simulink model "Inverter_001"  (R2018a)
settings: Solver=FixedStepDiscrete  StartTime=0.0  StopTime=inf  RelTol=1e-3  EnableMultiTasking=on
PreLoadFcn:
  | Sample_Time
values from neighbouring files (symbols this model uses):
  C_filt = 9.2e-6    (= 9.2e-06)    [master5.m]    (also in Sample_Time.m = 1.175e-06)
  Kcp = 5 /2    (= 2.5)    [master5.m]    (also in Parametri_final.m = Kcp_rac*20; Sample_Time.m = 8.8)
  Kcp0 = 5 /2    (= 2.5)    [master5.m]    (also in Parametri_final.m = Kc0p_rac*20; Sample_Time.m = 8.8)
  Kvp = 1    [master5.m]    (also in Parametri_final.m = 0.06652; Sample_Time.m = 2.4)
  Kvp0 = 1    [master5.m]    (also in Parametri_final.m = 0.06652; Sample_Time.m = 2.4)
  L_filt = 1e-3    (= 0.001)    [master5.m]    (also in Sample_Time.m = 0.01)
  Tcontrol = 5e-5     *2    (= 0.0001)    [Sample_Time.m]
  Tmeasure = 5e-5    (= 5e-05)    [Sample_Time.m]
  w = 2*pi*50    (= 314.159265359)    [master5.m]    (also in Parametri_final.m = 314.1592)
undefined symbols (not defined in the file or in its folder): A, ADCIN0, ADCIN1, ADCINA0, ADCINB0, bit, C_filtEST, CC_Tci, CC_Tci0, CC_Tcr, Compare, Control, conversion, DCAEVT1, DCAEVT1FILT, Digital, Down, ended, Event, Filtered, GPTRIP1SEL, GPTRIP2SEL, input, Module, of, Single, start, Trip, TZ1, TZ2, Up, VC_Tci, VC_Tci0, VC_Tcr, version, Zone
libraries: tiiqmathlib x92, etargetslib x20, c2802xlib x13, c2837xDlib x7, c28xdmclib x1
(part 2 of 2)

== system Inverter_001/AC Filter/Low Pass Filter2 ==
  Input : Inport
  TimeConstant : Inport  Port=2
  IQN1 x IQN2 : tiiqmathlib/IQN1 x IQN2  Q=10
  Sum1 : Sum  Inputs=|+-  AccumDataTypeStr=single
  Sum2 : Sum  Inputs=|++  AccumDataTypeStr=single
  Sum3 : Sum  Inputs=|+-
  Unit Delay : UnitDelay  SampleTime=-1
  Unit Delay1 : UnitDelay  SampleTime=-1
  Output : Outport
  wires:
  Input/1 -> Sum3/1, Sum1/1
  IQN1 x IQN2/1 -> Sum1/2  "TcState"
  Sum1/1 -> Sum3/2, Unit Delay/1  "HighPassFilterOutput"
  Sum2/1 -> Unit Delay1/1, IQN1 x IQN2/2  "state"
  Unit Delay/1 -> Sum2/1
  TimeConstant/1 -> IQN1 x IQN2/1  "tc"
  Unit Delay1/1 -> Sum2/2
  Sum3/1 -> Output/1  "HighPassFilterOutput"

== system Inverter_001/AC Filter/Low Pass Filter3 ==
  Input : Inport
  TimeConstant : Inport  Port=2
  IQN1 x IQN2 : tiiqmathlib/IQN1 x IQN2  Q=10
  Sum1 : Sum  Inputs=|+-  AccumDataTypeStr=single
  Sum2 : Sum  Inputs=|++  AccumDataTypeStr=single
  Sum3 : Sum  Inputs=|+-
  Unit Delay : UnitDelay  SampleTime=-1
  Unit Delay1 : UnitDelay  SampleTime=-1
  Output : Outport
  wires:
  Sum3/1 -> Output/1  "HighPassFilterOutput"
  Unit Delay1/1 -> Sum2/2
  TimeConstant/1 -> IQN1 x IQN2/1  "tc"
  Unit Delay/1 -> Sum2/1
  Sum2/1 -> IQN1 x IQN2/2, Unit Delay1/1  "state"
  Sum1/1 -> Unit Delay/1, Sum3/2  "HighPassFilterOutput"
  IQN1 x IQN2/1 -> Sum1/2  "TcState"
  Input/1 -> Sum1/1, Sum3/1

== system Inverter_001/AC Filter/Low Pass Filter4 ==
  Input : Inport
  TimeConstant : Inport  Port=2
  IQN1 x IQN2 : tiiqmathlib/IQN1 x IQN2  Q=10
  Sum1 : Sum  Inputs=|+-  AccumDataTypeStr=single
  Sum2 : Sum  Inputs=|++  AccumDataTypeStr=single
  Sum3 : Sum  Inputs=|+-
  Unit Delay : UnitDelay  SampleTime=-1
  Unit Delay1 : UnitDelay  SampleTime=-1
  Output : Outport
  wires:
  Input/1 -> Sum3/1, Sum1/1
  IQN1 x IQN2/1 -> Sum1/2  "TcState"
  Sum1/1 -> Sum3/2, Unit Delay/1  "HighPassFilterOutput"
  Sum2/1 -> Unit Delay1/1, IQN1 x IQN2/2  "state"
  Unit Delay/1 -> Sum2/1
  TimeConstant/1 -> IQN1 x IQN2/1  "tc"
  Unit Delay1/1 -> Sum2/2
  Sum3/1 -> Output/1  "HighPassFilterOutput"

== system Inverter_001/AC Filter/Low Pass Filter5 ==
  Input : Inport
  TimeConstant : Inport  Port=2
  IQN1 x IQN2 : tiiqmathlib/IQN1 x IQN2  Q=10
  Sum1 : Sum  Inputs=|+-  AccumDataTypeStr=single
  Sum2 : Sum  Inputs=|++  AccumDataTypeStr=single
  Sum3 : Sum  Inputs=|+-
  Unit Delay : UnitDelay  SampleTime=-1
  Unit Delay1 : UnitDelay  SampleTime=-1
  Output : Outport
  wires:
  Sum3/1 -> Output/1  "HighPassFilterOutput"
  Unit Delay1/1 -> Sum2/2
  TimeConstant/1 -> IQN1 x IQN2/1  "tc"
  Unit Delay/1 -> Sum2/1
  Sum2/1 -> IQN1 x IQN2/2, Unit Delay1/1  "state"
  Sum1/1 -> Unit Delay/1, Sum3/2  "HighPassFilterOutput"
  IQN1 x IQN2/1 -> Sum1/2  "TcState"
  Input/1 -> Sum1/1, Sum3/1

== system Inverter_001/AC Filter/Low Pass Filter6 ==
  Input : Inport
  TimeConstant : Inport  Port=2
  IQN1 x IQN2 : tiiqmathlib/IQN1 x IQN2  Q=10
  Sum1 : Sum  Inputs=|+-  AccumDataTypeStr=single
  Sum2 : Sum  Inputs=|++  AccumDataTypeStr=single
  Sum3 : Sum  Inputs=|+-
  Unit Delay : UnitDelay  SampleTime=-1
  Unit Delay1 : UnitDelay  SampleTime=-1
  Output : Outport
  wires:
  Input/1 -> Sum3/1, Sum1/1
  IQN1 x IQN2/1 -> Sum1/2  "TcState"
  Sum1/1 -> Sum3/2, Unit Delay/1  "HighPassFilterOutput"
  Sum2/1 -> Unit Delay1/1, IQN1 x IQN2/2  "state"
  Unit Delay/1 -> Sum2/1
  TimeConstant/1 -> IQN1 x IQN2/1  "tc"
  Unit Delay1/1 -> Sum2/2
  Sum3/1 -> Output/1  "HighPassFilterOutput"

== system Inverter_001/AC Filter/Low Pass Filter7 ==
  Input : Inport
  TimeConstant : Inport  Port=2
  IQN1 x IQN2 : tiiqmathlib/IQN1 x IQN2  Q=10
  Sum1 : Sum  Inputs=|+-  AccumDataTypeStr=single
  Sum2 : Sum  Inputs=|++  AccumDataTypeStr=single
  Sum3 : Sum  Inputs=|+-
  Unit Delay : UnitDelay  SampleTime=-1
  Unit Delay1 : UnitDelay  SampleTime=-1
  Output : Outport
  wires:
  Sum3/1 -> Output/1  "HighPassFilterOutput"
  Unit Delay1/1 -> Sum2/2
  TimeConstant/1 -> IQN1 x IQN2/1  "tc"
  Unit Delay/1 -> Sum2/1
  Sum2/1 -> IQN1 x IQN2/2, Unit Delay1/1  "state"
  Sum1/1 -> Unit Delay/1, Sum3/2  "HighPassFilterOutput"
  IQN1 x IQN2/1 -> Sum1/2  "TcState"
  Input/1 -> Sum1/1, Sum3/1

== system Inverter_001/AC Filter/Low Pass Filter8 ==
  Input : Inport
  TimeConstant : Inport  Port=2
  IQN1 x IQN2 : tiiqmathlib/IQN1 x IQN2  Q=10
  Sum1 : Sum  Inputs=|+-  AccumDataTypeStr=single
  Sum2 : Sum  Inputs=|++  AccumDataTypeStr=single
  Sum3 : Sum  Inputs=|+-
  Unit Delay : UnitDelay  SampleTime=-1
  Unit Delay1 : UnitDelay  SampleTime=-1
  Output : Outport
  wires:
  Input/1 -> Sum3/1, Sum1/1
  IQN1 x IQN2/1 -> Sum1/2  "TcState"
  Sum1/1 -> Sum3/2, Unit Delay/1  "HighPassFilterOutput"
  Sum2/1 -> Unit Delay1/1, IQN1 x IQN2/2  "state"
  Unit Delay/1 -> Sum2/1
  TimeConstant/1 -> IQN1 x IQN2/1  "tc"
  Unit Delay1/1 -> Sum2/2
  Sum3/1 -> Output/1  "HighPassFilterOutput"

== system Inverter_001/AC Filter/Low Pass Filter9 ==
  Input : Inport
  TimeConstant : Inport  Port=2
  IQN1 x IQN2 : tiiqmathlib/IQN1 x IQN2  Q=10
  Sum1 : Sum  Inputs=|+-  AccumDataTypeStr=single
  Sum2 : Sum  Inputs=|++  AccumDataTypeStr=single
  Sum3 : Sum  Inputs=|+-
  Unit Delay : UnitDelay  SampleTime=-1
  Unit Delay1 : UnitDelay  SampleTime=-1
  Output : Outport
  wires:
  Sum3/1 -> Output/1  "HighPassFilterOutput"
  Unit Delay1/1 -> Sum2/2
  TimeConstant/1 -> IQN1 x IQN2/1  "tc"
  Unit Delay/1 -> Sum2/1
  Sum2/1 -> IQN1 x IQN2/2, Unit Delay1/1  "state"
  Sum1/1 -> Unit Delay/1, Sum3/2  "HighPassFilterOutput"
  IQN1 x IQN2/1 -> Sum1/2  "TcState"
  Input/1 -> Sum1/1, Sum3/1

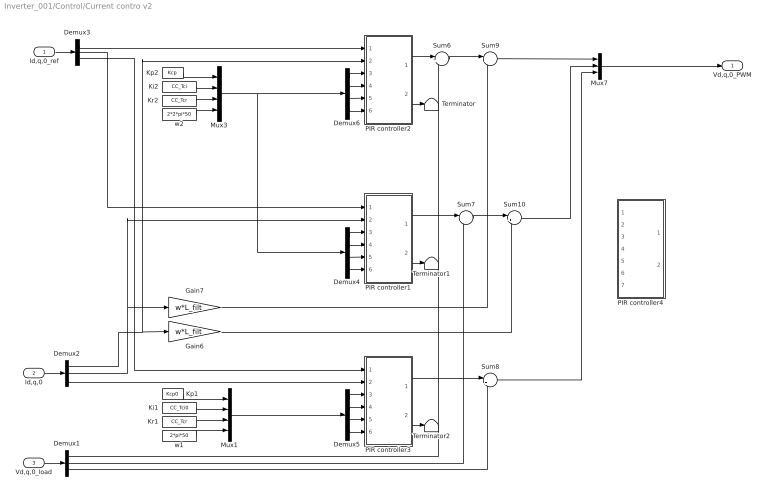
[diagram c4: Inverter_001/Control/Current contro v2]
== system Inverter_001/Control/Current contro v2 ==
  Id,q,0_ref : Inport
  Id,q,0 : Inport  Port=2
  Vd,q,0_load : Inport  Port=3
  Demux1 : Demux  Outputs=3
  Demux2 : Demux  Outputs=3
  Demux3 : Demux  Outputs=3
  Demux4 : Demux
  Demux5 : Demux
  Demux6 : Demux
  Gain6 : Gain  Gain=w*L_filt
  Gain7 : Gain  Gain=w*L_filt
  Ki1 : Constant  Value=CC_Tci0  OutDataTypeStr=fixdt(1,32,2^-10,0)  SampleTime=-1
  Ki2 : Constant  Value=CC_Tci  OutDataTypeStr=fixdt(1,32,2^-10,0)  SampleTime=-1
  Kp1 : Constant  Value=Kcp0  OutDataTypeStr=fixdt(1,32,2^-10,0)  SampleTime=-1
  Kp2 : Constant  Value=Kcp  OutDataTypeStr=fixdt(1,32,2^-10,0)  SampleTime=-1
  Kr1 : Constant  Value=CC_Tcr  OutDataTypeStr=fixdt(1,32,2^-10,0)  SampleTime=-1
  Kr2 : Constant  Value=CC_Tcr  OutDataTypeStr=fixdt(1,32,2^-10,0)  SampleTime=-1
  Mux1 : Mux
  Mux3 : Mux
  Mux7 : Mux  Inputs=3
  PIR controller1 : Subsystem
  PIR controller2 : Subsystem
  PIR controller3 : Subsystem
  PIR controller4 : Subsystem  Commented=on
  Sum{6..8,10} (4 alike) : Sum  Inputs=|++
  Sum9 : Sum  Inputs=|+-
  Terminator : Terminator
  Terminator1 : Terminator
  Terminator2 : Terminator
  w1 : Constant  Value=2*pi*50  OutDataTypeStr=fixdt(1,32,2^-10,0)  SampleTime=-1
  w2 : Constant  Value=2*2*pi*50  OutMin=[1e-4]  OutMax=[1000]  OutDataTypeStr=fixdt(1,32,2^-10,0)  SampleTime=-1
  Vd,q,0_PWM : Outport
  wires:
  Mux3/1 -> Demux4/1, Demux6/1
  w2/1 -> Mux3/4
  Kr2/1 -> Mux3/3
  Ki2/1 -> Mux3/2
  Kp2/1 -> Mux3/1
  Demux6/4 -> PIR controller2/6(w)
  Demux6/3 -> PIR controller2/5(Tr)
  Demux6/1 -> PIR controller2/3(Kp)
  Demux6/2 -> PIR controller2/4(Ti)
  Sum8/1 -> Mux7/3
  PIR controller1/1(Out1) -> Sum7/1
  Demux1/3 -> Sum8/2
  Demux3/3 -> PIR controller3/1(Reference)
  Demux2/3 -> PIR controller3/2(Measurement)
  PIR controller3/1(Out1) -> Sum8/1
  PIR controller2/1(Out1) -> Sum6/1
  Demux1/1 -> Sum6/2
  Demux1/2 -> Sum7/2
  Sum6/1 -> Sum9/1
  Sum9/1 -> Mux7/1
  Sum7/1 -> Sum10/1
  Sum10/1 -> Mux7/2
  Gain6/1 -> Sum10/2
  Gain7/1 -> Sum9/2
  Demux3/1 -> PIR controller2/1(Reference)
  Demux3/2 -> PIR controller1/1(Reference)
  Id,q,0/1 -> Demux2/1
  Id,q,0_ref/1 -> Demux3/1
  Vd,q,0_load/1 -> Demux1/1
  Demux2/2 -> PIR controller1/2(Measurement), Gain7/1
  Demux2/1 -> PIR controller2/2(Measurement), Gain6/1
  Demux5/1 -> PIR controller3/3(Kp)
  Demux5/2 -> PIR controller3/4(Ti)
  Demux5/3 -> PIR controller3/5(Tr)
  w1/1 -> Mux1/4
  Ki1/1 -> Mux1/2
  Kr1/1 -> Mux1/3
  Kp1/1 -> Mux1/1
  Mux1/1 -> Demux5/1
  Mux7/1 -> Vd,q,0_PWM/1
  Demux5/4 -> PIR controller3/6(w)
  Demux4/1 -> PIR controller1/3(Kp)
  Demux4/4 -> PIR controller1/6(w)
  Demux4/2 -> PIR controller1/4(Ti)
  Demux4/3 -> PIR controller1/5(Tr)
  PIR controller2/2(Error) -> Terminator/1
  PIR controller1/2(Error) -> Terminator1/1
  PIR controller3/2(Error) -> Terminator2/1

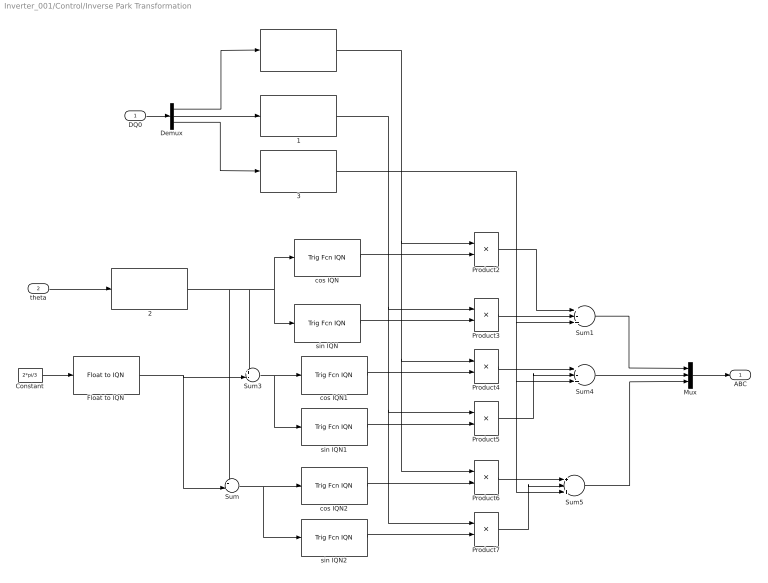
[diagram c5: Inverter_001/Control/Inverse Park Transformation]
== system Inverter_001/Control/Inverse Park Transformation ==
  DQ0 : Inport
  theta : Inport  Port=2
   {,1..3} (4 alike) : etargetslib/ 
  Constant : Constant  Value=2*pi/3  OutDataTypeStr=single
  Demux : Demux  Outputs=3
  Float to IQN : tiiqmathlib/Float to IQN  Q_value=10
  Mux : Mux  Inputs=3
  Product{2..7} (6 alike) : Product
  Sum : Sum  Inputs=++|
  Sum1 : Sum  Inputs=+-+
  Sum3 : Sum  Inputs=+-|
  Sum4 : Sum  Inputs=+-+
  Sum5 : Sum  Inputs=+-+
  cos IQN : tiiqmathlib/Trig Fcn IQN  functionOption=_IQcos
  cos IQN1 : tiiqmathlib/Trig Fcn IQN  functionOption=_IQcos
  cos IQN2 : tiiqmathlib/Trig Fcn IQN  functionOption=_IQcos
  sin IQN : tiiqmathlib/Trig Fcn IQN  functionOption=_IQsin
  sin IQN1 : tiiqmathlib/Trig Fcn IQN  functionOption=_IQsin
  sin IQN2 : tiiqmathlib/Trig Fcn IQN  functionOption=_IQsin
  ABC : Outport
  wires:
  " 2"/1 -> sin IQN/1, cos IQN/1, Sum3/1, Sum/1
  " 1"/1 -> Product7/1, Product5/1, Product3/1
  Mux/1 -> ABC/1
  Product2/1 -> Sum1/1
  Product3/1 -> Sum1/2
  sin IQN/1 -> Product3/2
  cos IQN/1 -> Product2/2
  Demux/2 -> " 1"/1
  Demux/1 -> " "/1
  theta/1 -> " 2"/1
  Demux/3 -> " 3"/1
  Constant/1 -> Float to IQN/1
  Float to IQN/1 -> Sum/2, Sum3/2
  " 3"/1 -> Sum5/3, Sum4/3, Sum1/3
  Sum3/1 -> sin IQN1/1, cos IQN1/1
  cos IQN1/1 -> Product4/2
  sin IQN1/1 -> Product5/2
  Product4/1 -> Sum4/1
  Product5/1 -> Sum4/2
  Sum4/1 -> Mux/2
  Sum/1 -> sin IQN2/1, cos IQN2/1
  " "/1 -> Product2/1, Product4/1, Product6/1
  cos IQN2/1 -> Product6/2
  sin IQN2/1 -> Product7/2
  Product6/1 -> Sum5/1
  Product7/1 -> Sum5/2
  Sum5/1 -> Mux/3
  DQ0/1 -> Demux/1
  Sum1/1 -> Mux/1

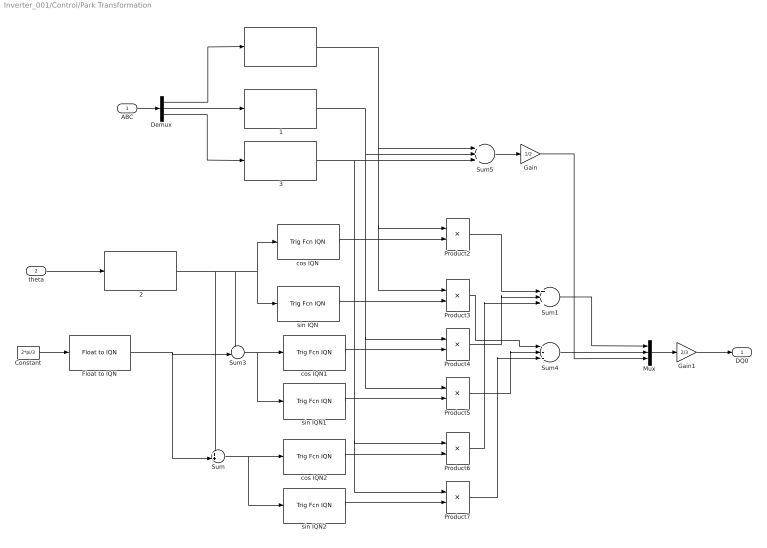
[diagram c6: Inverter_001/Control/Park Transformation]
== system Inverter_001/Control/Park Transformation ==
  ABC : Inport
  theta : Inport  Port=2
   {,1..3} (4 alike) : etargetslib/ 
  Constant : Constant  Value=2*pi/3  OutDataTypeStr=single
  Demux : Demux  Outputs=3
  Float to IQN : tiiqmathlib/Float to IQN  Q_value=10
  Gain : Gain  Gain=1/2  OutDataTypeStr=Inherit: Inherit via back propagation
  Gain1 : Gain  Gain=2/3  OutDataTypeStr=Inherit: Inherit via back propagation
  Mux : Mux  Inputs=3
  Product{2..7} (6 alike) : Product
  Sum : Sum  Inputs=++|
  Sum1 : Sum  Inputs=+++
  Sum3 : Sum  Inputs=+-|
  Sum4 : Sum  Inputs=---
  Sum5 : Sum  Inputs=+++
  cos IQN : tiiqmathlib/Trig Fcn IQN  functionOption=_IQcos
  cos IQN1 : tiiqmathlib/Trig Fcn IQN  functionOption=_IQcos
  cos IQN2 : tiiqmathlib/Trig Fcn IQN  functionOption=_IQcos
  sin IQN : tiiqmathlib/Trig Fcn IQN  functionOption=_IQsin
  sin IQN1 : tiiqmathlib/Trig Fcn IQN  functionOption=_IQsin
  sin IQN2 : tiiqmathlib/Trig Fcn IQN  functionOption=_IQsin
  DQ0 : Outport
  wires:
  Sum1/1 -> Mux/1
  ABC/1 -> Demux/1
  Sum5/1 -> Gain/1
  sin IQN2/1 -> Product7/2
  cos IQN2/1 -> Product6/2
  " "/1 -> Sum5/1, Product2/1, Product3/1
  Sum/1 -> cos IQN2/1, sin IQN2/1
  Sum4/1 -> Mux/2
  sin IQN1/1 -> Product5/2
  cos IQN1/1 -> Product4/2
  Sum3/1 -> cos IQN1/1, sin IQN1/1
  Float to IQN/1 -> Sum3/2, Sum/2
  Constant/1 -> Float to IQN/1
  Demux/3 -> " 3"/1
  theta/1 -> " 2"/1
  Demux/1 -> " "/1
  Demux/2 -> " 1"/1
  cos IQN/1 -> Product2/2
  sin IQN/1 -> Product3/2
  Mux/1 -> Gain1/1
  " 1"/1 -> Sum5/2, Product5/1, Product4/1
  " 2"/1 -> Sum/1, Sum3/1, cos IQN/1, sin IQN/1
  Product2/1 -> Sum1/1
  Product4/1 -> Sum1/2
  Product6/1 -> Sum1/3
  Product3/1 -> Sum4/1
  Product5/1 -> Sum4/2
  Product7/1 -> Sum4/3
  " 3"/1 -> Sum5/3, Product7/1, Product6/1
  Gain/1 -> Mux/3
  Gain1/1 -> DQ0/1

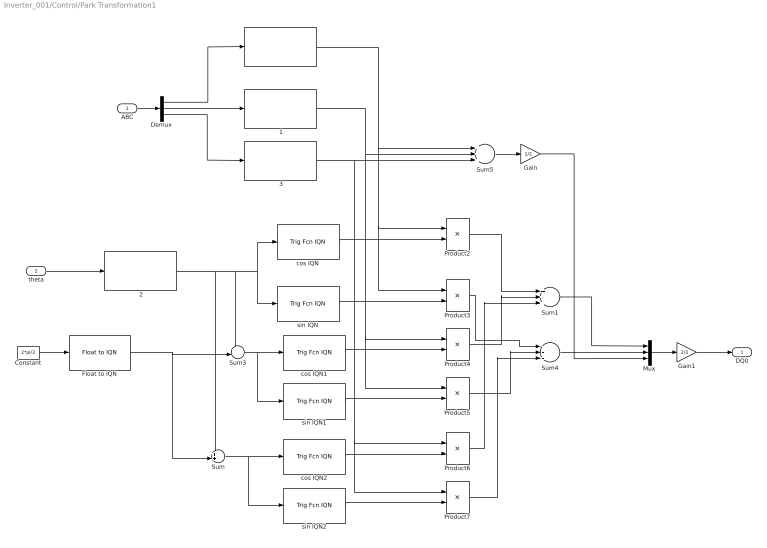
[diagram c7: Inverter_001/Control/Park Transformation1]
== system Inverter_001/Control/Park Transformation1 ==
  ABC : Inport
  theta : Inport  Port=2
   {,1..3} (4 alike) : etargetslib/ 
  Constant : Constant  Value=2*pi/3  OutDataTypeStr=single
  Demux : Demux  Outputs=3
  Float to IQN : tiiqmathlib/Float to IQN  Q_value=10
  Gain : Gain  Gain=1/2  OutDataTypeStr=Inherit: Inherit via back propagation
  Gain1 : Gain  Gain=2/3  OutDataTypeStr=Inherit: Inherit via back propagation
  Mux : Mux  Inputs=3
  Product{2..7} (6 alike) : Product
  Sum : Sum  Inputs=++|
  Sum1 : Sum  Inputs=+++
  Sum3 : Sum  Inputs=+-|
  Sum4 : Sum  Inputs=---
  Sum5 : Sum  Inputs=+++
  cos IQN : tiiqmathlib/Trig Fcn IQN  functionOption=_IQcos
  cos IQN1 : tiiqmathlib/Trig Fcn IQN  functionOption=_IQcos
  cos IQN2 : tiiqmathlib/Trig Fcn IQN  functionOption=_IQcos
  sin IQN : tiiqmathlib/Trig Fcn IQN  functionOption=_IQsin
  sin IQN1 : tiiqmathlib/Trig Fcn IQN  functionOption=_IQsin
  sin IQN2 : tiiqmathlib/Trig Fcn IQN  functionOption=_IQsin
  DQ0 : Outport
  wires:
  Gain1/1 -> DQ0/1
  Gain/1 -> Mux/3
  " 3"/1 -> Product6/1, Product7/1, Sum5/3
  Product7/1 -> Sum4/3
  Product5/1 -> Sum4/2
  Product3/1 -> Sum4/1
  Product6/1 -> Sum1/3
  Product4/1 -> Sum1/2
  Product2/1 -> Sum1/1
  " 2"/1 -> sin IQN/1, cos IQN/1, Sum3/1, Sum/1
  " 1"/1 -> Product4/1, Product5/1, Sum5/2
  Mux/1 -> Gain1/1
  sin IQN/1 -> Product3/2
  cos IQN/1 -> Product2/2
  Demux/2 -> " 1"/1
  Demux/1 -> " "/1
  theta/1 -> " 2"/1
  Demux/3 -> " 3"/1
  Constant/1 -> Float to IQN/1
  Float to IQN/1 -> Sum/2, Sum3/2
  Sum3/1 -> sin IQN1/1, cos IQN1/1
  cos IQN1/1 -> Product4/2
  sin IQN1/1 -> Product5/2
  Sum4/1 -> Mux/2
  Sum/1 -> sin IQN2/1, cos IQN2/1
  " "/1 -> Product3/1, Product2/1, Sum5/1
  cos IQN2/1 -> Product6/2
  sin IQN2/1 -> Product7/2
  Sum5/1 -> Gain/1
  ABC/1 -> Demux/1
  Sum1/1 -> Mux/1

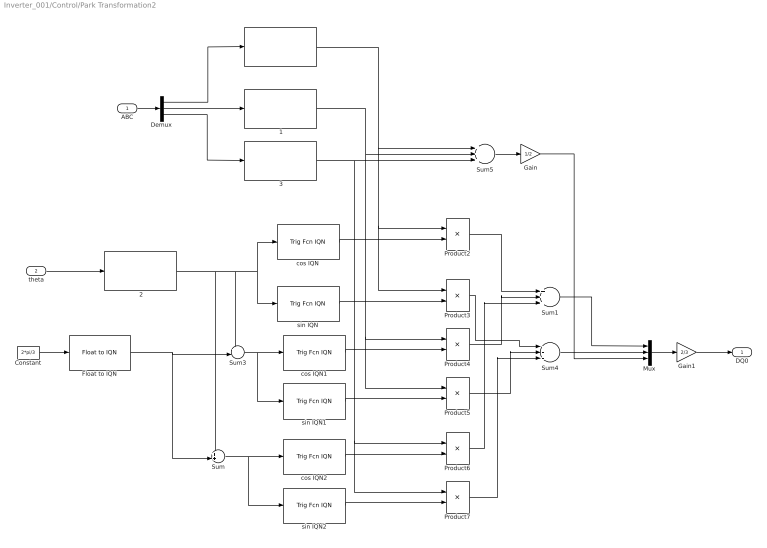
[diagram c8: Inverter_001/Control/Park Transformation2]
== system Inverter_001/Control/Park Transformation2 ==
  ABC : Inport
  theta : Inport  Port=2
   {,1..3} (4 alike) : etargetslib/ 
  Constant : Constant  Value=2*pi/3  OutDataTypeStr=single
  Demux : Demux  Outputs=3
  Float to IQN : tiiqmathlib/Float to IQN  Q_value=10
  Gain : Gain  Gain=1/2  OutDataTypeStr=Inherit: Inherit via back propagation
  Gain1 : Gain  Gain=2/3  OutDataTypeStr=Inherit: Inherit via back propagation
  Mux : Mux  Inputs=3
  Product{2..7} (6 alike) : Product
  Sum : Sum  Inputs=++|
  Sum1 : Sum  Inputs=+++
  Sum3 : Sum  Inputs=+-|
  Sum4 : Sum  Inputs=---
  Sum5 : Sum  Inputs=+++
  cos IQN : tiiqmathlib/Trig Fcn IQN  functionOption=_IQcos
  cos IQN1 : tiiqmathlib/Trig Fcn IQN  functionOption=_IQcos
  cos IQN2 : tiiqmathlib/Trig Fcn IQN  functionOption=_IQcos
  sin IQN : tiiqmathlib/Trig Fcn IQN  functionOption=_IQsin
  sin IQN1 : tiiqmathlib/Trig Fcn IQN  functionOption=_IQsin
  sin IQN2 : tiiqmathlib/Trig Fcn IQN  functionOption=_IQsin
  DQ0 : Outport
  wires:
  Sum1/1 -> Mux/1
  ABC/1 -> Demux/1
  Sum5/1 -> Gain/1
  sin IQN2/1 -> Product7/2
  cos IQN2/1 -> Product6/2
  " "/1 -> Sum5/1, Product2/1, Product3/1
  Sum/1 -> cos IQN2/1, sin IQN2/1
  Sum4/1 -> Mux/2
  sin IQN1/1 -> Product5/2
  cos IQN1/1 -> Product4/2
  Sum3/1 -> cos IQN1/1, sin IQN1/1
  Float to IQN/1 -> Sum3/2, Sum/2
  Constant/1 -> Float to IQN/1
  Demux/3 -> " 3"/1
  theta/1 -> " 2"/1
  Demux/1 -> " "/1
  Demux/2 -> " 1"/1
  cos IQN/1 -> Product2/2
  sin IQN/1 -> Product3/2
  Mux/1 -> Gain1/1
  " 1"/1 -> Sum5/2, Product5/1, Product4/1
  " 2"/1 -> Sum/1, Sum3/1, cos IQN/1, sin IQN/1
  Product2/1 -> Sum1/1
  Product4/1 -> Sum1/2
  Product6/1 -> Sum1/3
  Product3/1 -> Sum4/1
  Product5/1 -> Sum4/2
  Product7/1 -> Sum4/3
  " 3"/1 -> Sum5/3, Product7/1, Product6/1
  Gain/1 -> Mux/3
  Gain1/1 -> DQ0/1

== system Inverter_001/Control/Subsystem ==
  I1 : Inport
  I2 : Inport  Port=2
  Demux5 : Demux  Outputs=3
  Demux7 : Demux  Outputs=3
  Mux1 : Mux  Inputs=2
  Mux6 : Mux  Inputs=2
  Mux7 : Mux  Inputs=2
  O1 : Outport
  O2 : Outport  Port=2
  O3 : Outport  Port=3
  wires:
  Demux5/2 -> Mux6/1
  Demux5/1 -> Mux1/1
  Mux7/1 -> O3/1
  I1/1 -> Demux5/1
  Mux1/1 -> O1/1
  Mux6/1 -> O2/1
  I2/1 -> Demux7/1
  Demux5/3 -> Mux7/1
  Demux7/3 -> Mux7/2
  Demux7/2 -> Mux6/2
  Demux7/1 -> Mux1/2

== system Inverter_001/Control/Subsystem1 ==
  I1 : Inport
  I2 : Inport  Port=2
  Demux5 : Demux  Outputs=3
  Demux7 : Demux  Outputs=3
  Mux1 : Mux  Inputs=2
  Mux6 : Mux  Inputs=2
  Mux7 : Mux  Inputs=2
  O1 : Outport
  O2 : Outport  Port=2
  O3 : Outport  Port=3
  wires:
  Demux5/2 -> Mux6/1
  Demux5/1 -> Mux1/1
  Mux7/1 -> O3/1
  I1/1 -> Demux5/1
  Mux1/1 -> O1/1
  Mux6/1 -> O2/1
  I2/1 -> Demux7/1
  Demux5/3 -> Mux7/1
  Demux7/3 -> Mux7/2
  Demux7/2 -> Mux6/2
  Demux7/1 -> Mux1/2

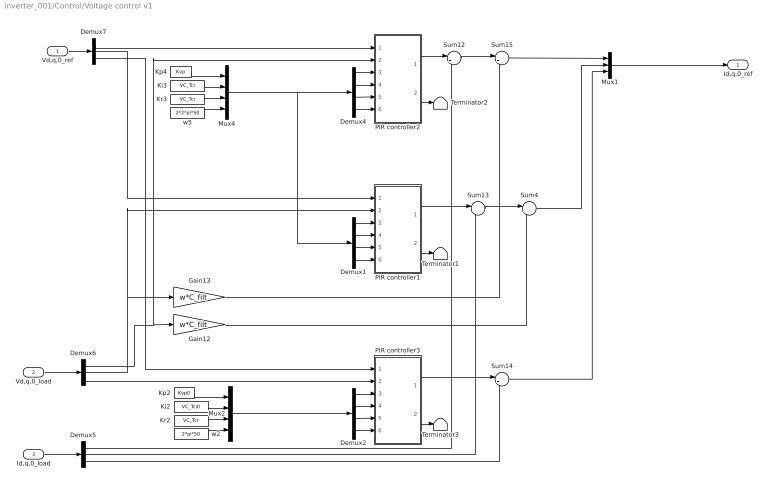
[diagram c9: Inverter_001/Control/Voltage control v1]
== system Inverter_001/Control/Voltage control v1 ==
  Vd,q,0_ref : Inport
  Vd,q,0_load : Inport  Port=2
  Id,q,0_load : Inport  Port=3
  Demux1 : Demux
  Demux2 : Demux
  Demux4 : Demux
  Demux5 : Demux  Outputs=3
  Demux6 : Demux  Outputs=3
  Demux7 : Demux  Outputs=3
  Gain12 : Gain  Gain=w*C_filt
  Gain13 : Gain  Gain=w*C_filt
  Ki2 : Constant  Value=VC_Tci0  OutDataTypeStr=fixdt(1,32,2^-10,0)  SampleTime=-1
  Ki3 : Constant  Value=VC_Tci  OutDataTypeStr=fixdt(1,32,2^-10,0)  SampleTime=-1
  Kp2 : Constant  Value=Kvp0  OutDataTypeStr=fixdt(1,32,2^-10,0)  SampleTime=-1
  Kp4 : Constant  Value=Kvp  OutDataTypeStr=fixdt(1,32,2^-10,0)  SampleTime=-1
  Kr2 : Constant  Value=VC_Tcr  OutDataTypeStr=fixdt(1,32,2^-10,0)  SampleTime=-1
  Kr3 : Constant  Value=VC_Tcr  OutDataTypeStr=fixdt(1,32,2^-10,0)  SampleTime=-1
  Mux1 : Mux  Inputs=3
  Mux2 : Mux
  Mux4 : Mux
  PIR controller1 : Subsystem
  PIR controller2 : Subsystem
  PIR controller3 : Subsystem
  Sum{4,12..14} (4 alike) : Sum  Inputs=|++
  Sum15 : Sum  Inputs=|+-
  Terminator1 : Terminator
  Terminator2 : Terminator
  Terminator3 : Terminator
  w2 : Constant  Value=2*pi*50  OutMin=[1e-4]  OutMax=[1000]  OutDataTypeStr=fixdt(1,32,2^-10,0)  SampleTime=-1
  w5 : Constant  Value=2*2*pi*50  OutMin=[1e-4]  OutMax=[1000]  OutDataTypeStr=fixdt(1,32,2^-10,0)  SampleTime=-1
  Id,q,0_ref : Outport
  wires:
  Vd,q,0_load/1 -> Demux6/1
  Vd,q,0_ref/1 -> Demux7/1
  Id,q,0_load/1 -> Demux5/1
  Demux6/1 -> PIR controller2/2(Measurement), Gain12/1
  Demux6/2 -> PIR controller1/2(Measurement), Gain13/1
  Demux7/2 -> PIR controller1/1(Reference)
  Demux7/1 -> PIR controller2/1(Reference)
  Gain13/1 -> Sum15/2
  Gain12/1 -> Sum4/2
  Sum4/1 -> Mux1/2
  Sum13/1 -> Sum4/1
  Sum15/1 -> Mux1/1
  Sum12/1 -> Sum15/1
  Demux5/2 -> Sum13/2
  Demux5/1 -> Sum12/2
  PIR controller2/1(Out1) -> Sum12/1
  PIR controller3/1(Out1) -> Sum14/1
  Demux6/3 -> PIR controller3/2(Measurement)
  Demux7/3 -> PIR controller3/1(Reference)
  Demux5/3 -> Sum14/2
  PIR controller1/1(Out1) -> Sum13/1
  Sum14/1 -> Mux1/3
  Mux1/1 -> Id,q,0_ref/1
  Mux4/1 -> Demux1/1, Demux4/1
  w5/1 -> Mux4/4
  Kr3/1 -> Mux4/3
  Ki3/1 -> Mux4/2
  Kp4/1 -> Mux4/1
  Demux4/4 -> PIR controller2/6(w)
  Demux4/3 -> PIR controller2/5(Tr)
  Demux4/1 -> PIR controller2/3(Kp)
  Demux4/2 -> PIR controller2/4(Ti)
  Demux1/4 -> PIR controller1/6(w)
  Demux1/3 -> PIR controller1/5(Tr)
  Demux1/1 -> PIR controller1/3(Kp)
  Demux1/2 -> PIR controller1/4(Ti)
  Demux2/4 -> PIR controller3/6(w)
  Demux2/3 -> PIR controller3/5(Tr)
  Demux2/2 -> PIR controller3/4(Ti)
  Demux2/1 -> PIR controller3/3(Kp)
  Mux2/1 -> Demux2/1
  w2/1 -> Mux2/4
  Kr2/1 -> Mux2/3
  Ki2/1 -> Mux2/2
  Kp2/1 -> Mux2/1
  PIR controller2/2(Error) -> Terminator2/1
  PIR controller1/2(Error) -> Terminator1/1
  PIR controller3/2(Error) -> Terminator3/1

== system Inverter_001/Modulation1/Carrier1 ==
  In1 : Inport
  Gain : Gain  Gain=-0.5
  Gain1 : Gain  Gain=-0.5
  MATLAB Function : MATLAB Function  Commented=on  TreatAsAtomicUnit=on
  MinMax : MinMax  ZeroCross=off
  MinMax1 : MinMax  Function=max  ZeroCross=off
  Sum : Sum  Inputs=|++
  Out1 : Outport
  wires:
  MinMax/1 -> MATLAB Function/1(In1), Gain/1
  MinMax1/1 -> MATLAB Function/2(In2), Gain1/1
  Gain/1 -> Sum/1
  Gain1/1 -> Sum/2
  In1/1 -> MinMax/1, MinMax1/1
  Sum/1 -> Out1/1

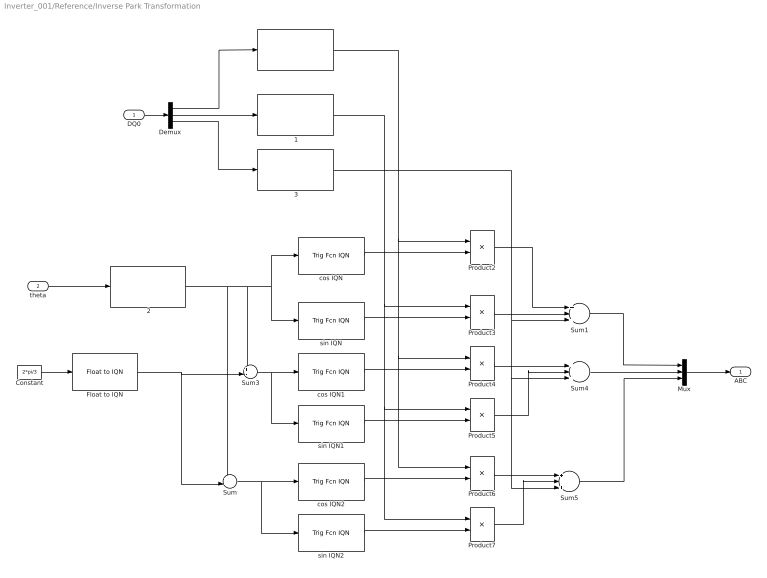
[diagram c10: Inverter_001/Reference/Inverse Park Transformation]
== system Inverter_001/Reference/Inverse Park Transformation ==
  DQ0 : Inport
  theta : Inport  Port=2
   {,1..3} (4 alike) : etargetslib/ 
  Constant : Constant  Value=2*pi/3  OutDataTypeStr=single
  Demux : Demux  Outputs=3
  Float to IQN : tiiqmathlib/Float to IQN  Q_value=10
  Mux : Mux  Inputs=3
  Product{2..7} (6 alike) : Product
  Sum : Sum  Inputs=++|
  Sum1 : Sum  Inputs=+-+
  Sum3 : Sum  Inputs=+-|
  Sum4 : Sum  Inputs=+-+
  Sum5 : Sum  Inputs=+-+
  cos IQN : tiiqmathlib/Trig Fcn IQN  functionOption=_IQcos
  cos IQN1 : tiiqmathlib/Trig Fcn IQN  functionOption=_IQcos
  cos IQN2 : tiiqmathlib/Trig Fcn IQN  functionOption=_IQcos
  sin IQN : tiiqmathlib/Trig Fcn IQN  functionOption=_IQsin
  sin IQN1 : tiiqmathlib/Trig Fcn IQN  functionOption=_IQsin
  sin IQN2 : tiiqmathlib/Trig Fcn IQN  functionOption=_IQsin
  ABC : Outport
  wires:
  " 2"/1 -> sin IQN/1, cos IQN/1, Sum3/1, Sum/1
  " 1"/1 -> Product7/1, Product5/1, Product3/1
  Product2/1 -> Sum1/1
  Product3/1 -> Sum1/2
  sin IQN/1 -> Product3/2
  cos IQN/1 -> Product2/2
  Demux/2 -> " 1"/1
  Demux/1 -> " "/1
  theta/1 -> " 2"/1
  Demux/3 -> " 3"/1
  Constant/1 -> Float to IQN/1
  Float to IQN/1 -> Sum/2, Sum3/2
  " 3"/1 -> Sum5/3, Sum4/3, Sum1/3
  Sum3/1 -> sin IQN1/1, cos IQN1/1
  cos IQN1/1 -> Product4/2
  sin IQN1/1 -> Product5/2
  Product4/1 -> Sum4/1
  Product5/1 -> Sum4/2
  Sum4/1 -> Mux/2
  Sum/1 -> sin IQN2/1, cos IQN2/1
  " "/1 -> Product2/1, Product4/1, Product6/1
  cos IQN2/1 -> Product6/2
  sin IQN2/1 -> Product7/2
  Product6/1 -> Sum5/1
  Product7/1 -> Sum5/2
  Sum5/1 -> Mux/3
  DQ0/1 -> Demux/1
  Sum1/1 -> Mux/1
  Mux/1 -> ABC/1

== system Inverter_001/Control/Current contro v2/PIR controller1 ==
  Reference : Inport
  Measurement : Inport  Port=2
  Kp : Inport  Port=3
  Ti : Inport  Port=4
  Tr : Inport  Port=5
  w : Inport  Port=6
  Data Type Conversion : DataTypeConversion  OutDataTypeStr=fixdt(1,32,2^-10,0)
  Gain : Gain  Gain=Control.Ts
  Gain1 : Gain  Gain=Control.Ts
  IQN1 x IQN{1..3,6..7} (5 alike) : tiiqmathlib/IQN1 x IQN2  Q=10
  Sum : Sum  Inputs=|+-
  Sum1 : Sum  Inputs=+++
  Sum11 : Sum  Inputs=|+-
  Sum3 : Sum  Inputs=|++
  Sum4 : Sum  Inputs=|++
  Sum5 : Sum  Inputs=|++
  Unit Delay{,1..3} (4 alike) : UnitDelay  SampleTime=-1
  Out1 : Outport
  Error : Outport  Port=2
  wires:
  Gain/1 -> Sum5/1
  Data Type Conversion/1 -> Sum5/2
  Tr/1 -> IQN1 x IQN1/2
  Gain1/1 -> Sum4/1
  Sum11/1 -> Gain/1
  Sum/1 -> Sum11/1, IQN1 x IQN2/1, Sum3/1, Error/1
  Ti/1 -> IQN1 x IQN3/2
  Sum1/1 -> Out1/1
  Unit Delay/1 -> Sum3/2
  Unit Delay1/1 -> Sum4/2
  Sum5/1 -> IQN1 x IQN1/1, Gain1/1, Unit Delay2/1
  Unit Delay2/1 -> Data Type Conversion/1
  Unit Delay3/1 -> Sum11/2
  Kp/1 -> IQN1 x IQN2/2
  IQN1 x IQN2/1 -> Sum1/2
  Sum3/1 -> IQN1 x IQN3/1, Unit Delay/1
  IQN1 x IQN7/1 -> IQN1 x IQN6/2
  w/1 -> IQN1 x IQN7/2, IQN1 x IQN7/1
  Reference/1 -> Sum/1
  Measurement/1 -> Sum/2
  Sum4/1 -> IQN1 x IQN6/1, Unit Delay1/1
  IQN1 x IQN3/1 -> Sum1/3
  IQN1 x IQN1/1 -> Sum1/1
  IQN1 x IQN6/1 -> Unit Delay3/1

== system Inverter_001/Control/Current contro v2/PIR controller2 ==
  Reference : Inport
  Measurement : Inport  Port=2
  Kp : Inport  Port=3
  Ti : Inport  Port=4
  Tr : Inport  Port=5
  w : Inport  Port=6
  Data Type Conversion : DataTypeConversion  OutDataTypeStr=fixdt(1,32,2^-10,0)
  Gain : Gain  Gain=Control.Ts
  Gain1 : Gain  Gain=Control.Ts
  IQN1 x IQN{1..3,6..7} (5 alike) : tiiqmathlib/IQN1 x IQN2  Q=10
  Sum : Sum  Inputs=|+-
  Sum1 : Sum  Inputs=+++
  Sum11 : Sum  Inputs=|+-
  Sum3 : Sum  Inputs=|++
  Sum4 : Sum  Inputs=|++
  Sum5 : Sum  Inputs=|++
  Unit Delay{,1..3} (4 alike) : UnitDelay  SampleTime=-1
  Out1 : Outport
  Error : Outport  Port=2
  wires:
  IQN1 x IQN6/1 -> Unit Delay3/1
  IQN1 x IQN1/1 -> Sum1/1
  IQN1 x IQN3/1 -> Sum1/3
  Sum4/1 -> Unit Delay1/1, IQN1 x IQN6/1
  Measurement/1 -> Sum/2
  Reference/1 -> Sum/1
  w/1 -> IQN1 x IQN7/1, IQN1 x IQN7/2
  IQN1 x IQN7/1 -> IQN1 x IQN6/2
  Sum3/1 -> Unit Delay/1, IQN1 x IQN3/1
  IQN1 x IQN2/1 -> Sum1/2
  Kp/1 -> IQN1 x IQN2/2
  Unit Delay3/1 -> Sum11/2
  Unit Delay2/1 -> Data Type Conversion/1
  Sum5/1 -> Unit Delay2/1, Gain1/1, IQN1 x IQN1/1
  Unit Delay1/1 -> Sum4/2
  Unit Delay/1 -> Sum3/2
  Sum1/1 -> Out1/1
  Ti/1 -> IQN1 x IQN3/2
  Sum/1 -> Error/1, Sum3/1, IQN1 x IQN2/1, Sum11/1
  Sum11/1 -> Gain/1
  Gain1/1 -> Sum4/1
  Tr/1 -> IQN1 x IQN1/2
  Data Type Conversion/1 -> Sum5/2
  Gain/1 -> Sum5/1

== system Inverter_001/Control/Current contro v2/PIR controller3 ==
  Reference : Inport
  Measurement : Inport  Port=2
  Kp : Inport  Port=3
  Ti : Inport  Port=4
  Tr : Inport  Port=5
  w : Inport  Port=6
  Data Type Conversion : DataTypeConversion  OutDataTypeStr=fixdt(1,32,2^-10,0)
  Gain : Gain  Gain=Control.Ts
  Gain1 : Gain  Gain=Control.Ts
  IQN1 x IQN{1..3,6..7} (5 alike) : tiiqmathlib/IQN1 x IQN2  Q=10
  Sum : Sum  Inputs=|+-
  Sum1 : Sum  Inputs=+++
  Sum11 : Sum  Inputs=|+-
  Sum3 : Sum  Inputs=|++
  Sum4 : Sum  Inputs=|++
  Sum5 : Sum  Inputs=|++
  Unit Delay{,1..3} (4 alike) : UnitDelay  SampleTime=-1
  Out1 : Outport
  Error : Outport  Port=2
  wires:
  IQN1 x IQN6/1 -> Unit Delay3/1
  IQN1 x IQN1/1 -> Sum1/1
  IQN1 x IQN3/1 -> Sum1/3
  Sum4/1 -> Unit Delay1/1, IQN1 x IQN6/1
  Measurement/1 -> Sum/2
  Reference/1 -> Sum/1
  w/1 -> IQN1 x IQN7/1, IQN1 x IQN7/2
  IQN1 x IQN7/1 -> IQN1 x IQN6/2
  Sum3/1 -> Unit Delay/1, IQN1 x IQN3/1
  IQN1 x IQN2/1 -> Sum1/2
  Kp/1 -> IQN1 x IQN2/2
  Unit Delay3/1 -> Sum11/2
  Unit Delay2/1 -> Data Type Conversion/1
  Sum5/1 -> Unit Delay2/1, Gain1/1, IQN1 x IQN1/1
  Unit Delay1/1 -> Sum4/2
  Unit Delay/1 -> Sum3/2
  Sum1/1 -> Out1/1
  Ti/1 -> IQN1 x IQN3/2
  Sum/1 -> Error/1, Sum3/1, IQN1 x IQN2/1, Sum11/1
  Sum11/1 -> Gain/1
  Gain1/1 -> Sum4/1
  Tr/1 -> IQN1 x IQN1/2
  Data Type Conversion/1 -> Sum5/2
  Gain/1 -> Sum5/1

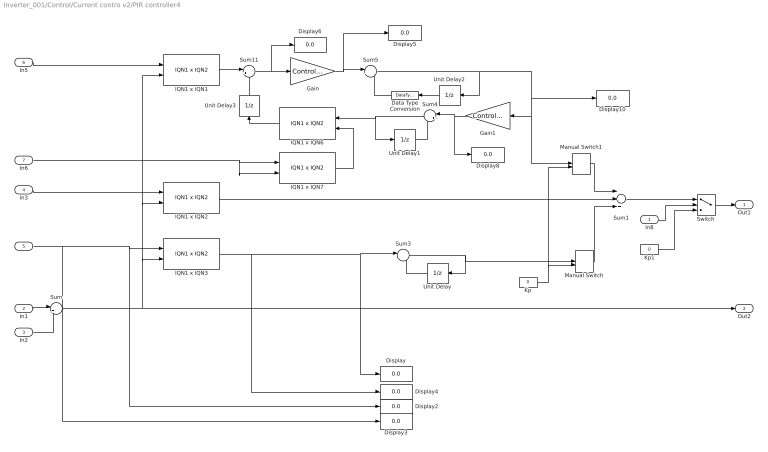
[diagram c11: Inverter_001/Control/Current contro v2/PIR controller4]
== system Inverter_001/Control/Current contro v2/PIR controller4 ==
  In8 : Inport
  In1 : Inport  Port=2
  In2 : Inport  Port=3
  In3 : Inport  Port=4
  Ti : Inport  Port=5
  In5 : Inport  Port=6
  In6 : Inport  Port=7
  Data Type Conversion : DataTypeConversion  OutDataTypeStr=fixdt(1,32,2^-10,0)
  Display{,2..6,8,10} (8 alike) : Display
  Gain : Gain  Gain=Control.Ts
  Gain1 : Gain  Gain=Control.Ts
  IQN1 x IQN{1..3,6..7} (5 alike) : tiiqmathlib/IQN1 x IQN2  Q=10
  Kp : Constant  Value=0  OutDataTypeStr=fixdt(1,32,2^-10,0)
  Kp1 : Constant  Value=0  OutDataTypeStr=fixdt(1,32,2^-10,0)
  Manual Switch : ManualSwitch
  Manual Switch1 : ManualSwitch
  Sum : Sum  Inputs=|+-
  Sum1 : Sum  Inputs=+++
  Sum11 : Sum  Inputs=|+-
  Sum3 : Sum  Inputs=|++
  Sum4 : Sum  Inputs=|++
  Sum5 : Sum  Inputs=|++
  Switch : Switch
  Unit Delay{,1..3} (4 alike) : UnitDelay  SampleTime=-1
  Out1 : Outport
  Out2 : Outport  Port=2
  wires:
  IQN1 x IQN6/1 -> Unit Delay3/1
  Manual Switch1/1 -> Sum1/1
  Manual Switch/1 -> Sum1/3
  Kp/1 -> Manual Switch/2, Manual Switch1/2
  Sum4/1 -> Unit Delay1/1, IQN1 x IQN6/1
  In2/1 -> Sum/2
  In1/1 -> Sum/1
  In6/1 -> IQN1 x IQN7/1, IQN1 x IQN7/2
  IQN1 x IQN7/1 -> IQN1 x IQN6/2
  Sum3/1 -> Unit Delay/1, Manual Switch/1
  IQN1 x IQN2/1 -> Sum1/2
  In3/1 -> IQN1 x IQN2/1
  Unit Delay3/1 -> Sum11/2
  Unit Delay2/1 -> Data Type Conversion/1
  Sum5/1 -> Unit Delay2/1, Manual Switch1/1, Gain1/1, Display10/1
  Unit Delay1/1 -> Sum4/2
  Unit Delay/1 -> Sum3/2
  In8/1 -> Switch/2
  Kp1/1 -> Switch/3
  Sum1/1 -> Switch/1
  Switch/1 -> Out1/1
  Ti/1 -> Display2/1, IQN1 x IQN3/1, Display3/1
  IQN1 x IQN1/1 -> Sum11/1
  IQN1 x IQN3/1 -> Display4/1, Display/1, Sum3/1
  Sum11/1 -> Display6/1, Gain/1
  Gain1/1 -> Display8/1, Sum4/1
  In5/1 -> IQN1 x IQN1/1
  Sum/1 -> IQN1 x IQN1/2, IQN1 x IQN2/2, IQN1 x IQN3/2, Out2/1
  Data Type Conversion/1 -> Sum5/2
  Gain/1 -> Display5/1, Sum5/1

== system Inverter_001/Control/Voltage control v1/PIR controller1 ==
  Reference : Inport
  Measurement : Inport  Port=2
  Kp : Inport  Port=3
  Ti : Inport  Port=4
  Tr : Inport  Port=5
  w : Inport  Port=6
  Data Type Conversion : DataTypeConversion  OutDataTypeStr=fixdt(1,32,2^-10,0)
  Gain : Gain  Gain=Control.Ts
  Gain1 : Gain  Gain=Control.Ts
  IQN1 x IQN{1..3,6..7} (5 alike) : tiiqmathlib/IQN1 x IQN2  Q=10
  Sum : Sum  Inputs=|+-
  Sum1 : Sum  Inputs=+++
  Sum11 : Sum  Inputs=|+-
  Sum3 : Sum  Inputs=|++
  Sum4 : Sum  Inputs=|++
  Sum5 : Sum  Inputs=|++
  Unit Delay{,1..3} (4 alike) : UnitDelay  SampleTime=-1
  Out1 : Outport
  Error : Outport  Port=2
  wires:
  Gain/1 -> Sum5/1
  Data Type Conversion/1 -> Sum5/2
  Tr/1 -> IQN1 x IQN1/2
  Gain1/1 -> Sum4/1
  Sum11/1 -> Gain/1
  Sum/1 -> Sum11/1, IQN1 x IQN2/1, Sum3/1, Error/1
  Ti/1 -> IQN1 x IQN3/2
  Sum1/1 -> Out1/1
  Unit Delay/1 -> Sum3/2
  Unit Delay1/1 -> Sum4/2
  Sum5/1 -> IQN1 x IQN1/1, Gain1/1, Unit Delay2/1
  Unit Delay2/1 -> Data Type Conversion/1
  Unit Delay3/1 -> Sum11/2
  Kp/1 -> IQN1 x IQN2/2
  IQN1 x IQN2/1 -> Sum1/2
  Sum3/1 -> IQN1 x IQN3/1, Unit Delay/1
  IQN1 x IQN7/1 -> IQN1 x IQN6/2
  w/1 -> IQN1 x IQN7/2, IQN1 x IQN7/1
  Reference/1 -> Sum/1
  Measurement/1 -> Sum/2
  Sum4/1 -> IQN1 x IQN6/1, Unit Delay1/1
  IQN1 x IQN3/1 -> Sum1/3
  IQN1 x IQN1/1 -> Sum1/1
  IQN1 x IQN6/1 -> Unit Delay3/1

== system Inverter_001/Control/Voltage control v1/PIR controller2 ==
  Reference : Inport
  Measurement : Inport  Port=2
  Kp : Inport  Port=3
  Ti : Inport  Port=4
  Tr : Inport  Port=5
  w : Inport  Port=6
  Data Type Conversion : DataTypeConversion  OutDataTypeStr=fixdt(1,32,2^-10,0)
  Gain : Gain  Gain=Control.Ts
  Gain1 : Gain  Gain=Control.Ts
  IQN1 x IQN{1..3,6..7} (5 alike) : tiiqmathlib/IQN1 x IQN2  Q=10
  Sum : Sum  Inputs=|+-
  Sum1 : Sum  Inputs=+++
  Sum11 : Sum  Inputs=|+-
  Sum3 : Sum  Inputs=|++
  Sum4 : Sum  Inputs=|++
  Sum5 : Sum  Inputs=|++
  Unit Delay{,1..3} (4 alike) : UnitDelay  SampleTime=-1
  Out1 : Outport
  Error : Outport  Port=2
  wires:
  IQN1 x IQN6/1 -> Unit Delay3/1
  IQN1 x IQN1/1 -> Sum1/1
  IQN1 x IQN3/1 -> Sum1/3
  Sum4/1 -> Unit Delay1/1, IQN1 x IQN6/1
  Measurement/1 -> Sum/2
  Reference/1 -> Sum/1
  w/1 -> IQN1 x IQN7/1, IQN1 x IQN7/2
  IQN1 x IQN7/1 -> IQN1 x IQN6/2
  Sum3/1 -> Unit Delay/1, IQN1 x IQN3/1
  IQN1 x IQN2/1 -> Sum1/2
  Kp/1 -> IQN1 x IQN2/2
  Unit Delay3/1 -> Sum11/2
  Unit Delay2/1 -> Data Type Conversion/1
  Sum5/1 -> Unit Delay2/1, Gain1/1, IQN1 x IQN1/1
  Unit Delay1/1 -> Sum4/2
  Unit Delay/1 -> Sum3/2
  Sum1/1 -> Out1/1
  Ti/1 -> IQN1 x IQN3/2
  Sum/1 -> Error/1, Sum3/1, IQN1 x IQN2/1, Sum11/1
  Sum11/1 -> Gain/1
  Gain1/1 -> Sum4/1
  Tr/1 -> IQN1 x IQN1/2
  Data Type Conversion/1 -> Sum5/2
  Gain/1 -> Sum5/1

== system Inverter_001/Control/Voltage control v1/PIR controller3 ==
  Reference : Inport
  Measurement : Inport  Port=2
  Kp : Inport  Port=3
  Ti : Inport  Port=4
  Tr : Inport  Port=5
  w : Inport  Port=6
  Data Type Conversion : DataTypeConversion  OutDataTypeStr=fixdt(1,32,2^-10,0)
  Gain : Gain  Gain=Control.Ts
  Gain1 : Gain  Gain=Control.Ts
  IQN1 x IQN{1..3,6..7} (5 alike) : tiiqmathlib/IQN1 x IQN2  Q=10
  Sum : Sum  Inputs=|+-
  Sum1 : Sum  Inputs=+++
  Sum11 : Sum  Inputs=|+-
  Sum3 : Sum  Inputs=|++
  Sum4 : Sum  Inputs=|++
  Sum5 : Sum  Inputs=|++
  Unit Delay{,1..3} (4 alike) : UnitDelay  SampleTime=-1
  Out1 : Outport
  Error : Outport  Port=2
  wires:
  IQN1 x IQN6/1 -> Unit Delay3/1
  IQN1 x IQN1/1 -> Sum1/1
  IQN1 x IQN3/1 -> Sum1/3
  Sum4/1 -> Unit Delay1/1, IQN1 x IQN6/1
  Measurement/1 -> Sum/2
  Reference/1 -> Sum/1
  w/1 -> IQN1 x IQN7/1, IQN1 x IQN7/2
  IQN1 x IQN7/1 -> IQN1 x IQN6/2
  Sum3/1 -> Unit Delay/1, IQN1 x IQN3/1
  IQN1 x IQN2/1 -> Sum1/2
  Kp/1 -> IQN1 x IQN2/2
  Unit Delay3/1 -> Sum11/2
  Unit Delay2/1 -> Data Type Conversion/1
  Sum5/1 -> Unit Delay2/1, Gain1/1, IQN1 x IQN1/1
  Unit Delay1/1 -> Sum4/2
  Unit Delay/1 -> Sum3/2
  Sum1/1 -> Out1/1
  Ti/1 -> IQN1 x IQN3/2
  Sum/1 -> Error/1, Sum3/1, IQN1 x IQN2/1, Sum11/1
  Sum11/1 -> Gain/1
  Gain1/1 -> Sum4/1
  Tr/1 -> IQN1 x IQN1/2
  Data Type Conversion/1 -> Sum5/2
  Gain/1 -> Sum5/1

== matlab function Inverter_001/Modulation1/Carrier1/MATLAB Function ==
function y = fcn(In1, In2)

temp_min = -0.5 * In1; % min
temp_max = -0.5 * In2; % max
temp_mid = temp_min + temp_max; % min

y = temp_mid;
